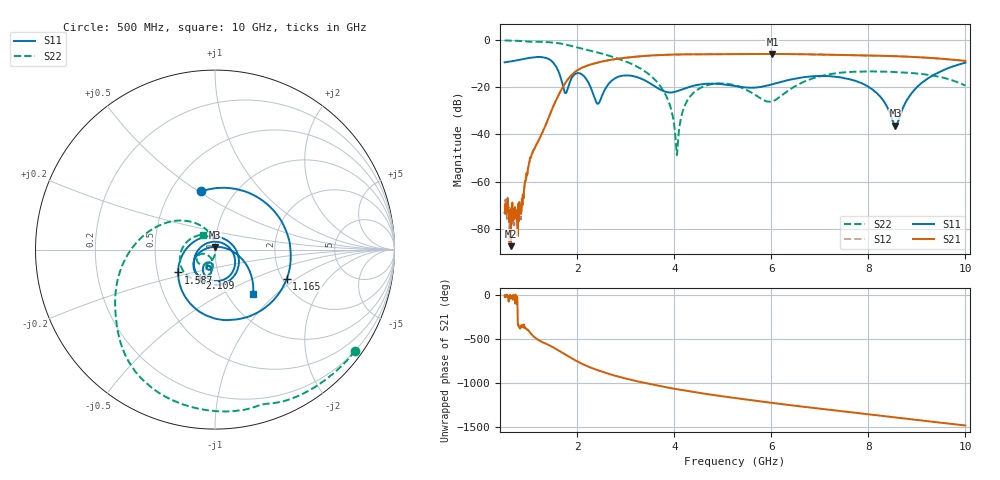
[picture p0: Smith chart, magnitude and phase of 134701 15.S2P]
!  2-Port S-parameters saved by WinCal
! VAR MeasName=S-Parameters (CALIBRATED_DATA) read from VNA (N5242A)
! VAR MeasDate=2013-7-3 16:29:55
! VAR NAME=134701 15
! VAR FILENAME=134701 15.S2P
! VAR DATE=2013-7-3 16:29:55
! VAR PHYS_PORTS=1,2
# Hz S MA R 50
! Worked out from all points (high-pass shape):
!   1601 points, 500 MHz to 10 GHz, reference 50 ohm
!   highest |S21| = -6.03 dB at 6.022 GHz (marker M1); lowest = -87.2 dB at 630.6 MHz (marker M2)
!   |S21| within 3 dB of the highest: 2.55 GHz to end of sweep
!   lowest |S11| = -36.4 dB at 8.557 GHz (marker M3), VSWR 1.03, Z = 49.9 + j1.51 ohm
!   |S11| at or under -10 dB: 1.514 GHz to 9.949 GHz (8.435 GHz wide, 147 % of centre)
!   |S22| runs from -48.7 to -0.3 dB; largest |S21 - S12| = 0.0027
!   S11 on the Smith chart (normalised r, x): 500 MHz: 0.70, +0.51; 1.165 GHz: 2.11, -0.84; 1.587 GHz: 0.64, -0.17; 2.109 GHz: 0.80, -0.26; 10 GHz: 1.31, -0.73
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5e8  0.333 103.1  0.0002237 -5.7  0.0003061 -19.0  0.9632 -35.9
6.30625e8  0.3482 81.5  4.376e-05 -22.7  0.0001935 -17.3  0.9555 -45.2
8.0875e8  0.3762 50.4  0.0002715 -6.8  0.0002445 -26.8  0.9414 -57.9
1.165e9  0.4314 -22.0  0.006389 -142.1  0.006435 -141.3  0.9064 -81.7
1.586562e9  0.2421 -148.3  0.05984 96.1  0.05972 95.8  0.8491 -113.8
1.75875e9  0.07394 76.0  0.1251 39.9  0.1247 39.9  0.79 -127.3
2.085312e9  0.1877 -110.2  0.2533 -62.0  0.2529 -62.1  0.6513 -148.5
2.109062e9  0.1801 -118.2  0.2598 -68.3  0.2594 -68.4  0.6428 -149.9
2.417812e9  0.04419 92.1  0.3291 -137.7  0.3283 -137.6  0.5367 -168.1
2.750312e9  0.147 -42.7  0.3849 163.9  0.3844 163.9  0.4269 172.7
3.670625e9  0.09327 -124.6  0.4733 44.9  0.4728 44.9  0.1182 112.9
3.908125e9  0.07669 -110.9  0.4833 20.0  0.4837 19.9  0.04144 93.3
4.050625e9  0.08138 -102.1  0.4877 5.8  0.4875 5.7  0.003663 2.6
4.383125e9  0.1055 -99.5  0.4921 -25.0  0.4921 -25.0  0.07365 -109.9
5.25e9  0.1051 -116.1  0.4957 -94.9  0.4962 -94.9  0.1084 -156.5
6.021875e9  0.1146 -99.7  0.4996 -150.6  0.4991 -150.7  0.05011 -122.7
6.835312e9  0.1683 -114.6  0.4897 154.0  0.4901 154.0  0.1506 -105.0
7.868438e9  0.1197 -157.0  0.4675 87.7  0.4675 87.6  0.2122 -139.3
8.420625e9  0.03218 158.5  0.4531 52.4  0.4517 52.4  0.2102 -155.4
8.557188e9  0.0152 93.9  0.4478 43.8  0.4477 43.8  0.2071 -159.2
9.067812e9  0.1152 -9.9  0.4241 10.8  0.4241 10.9  0.1907 -176.1
1e10  0.3272 -49.7  0.3565 -47.5  0.3578 -47.3  0.1072 128.4
